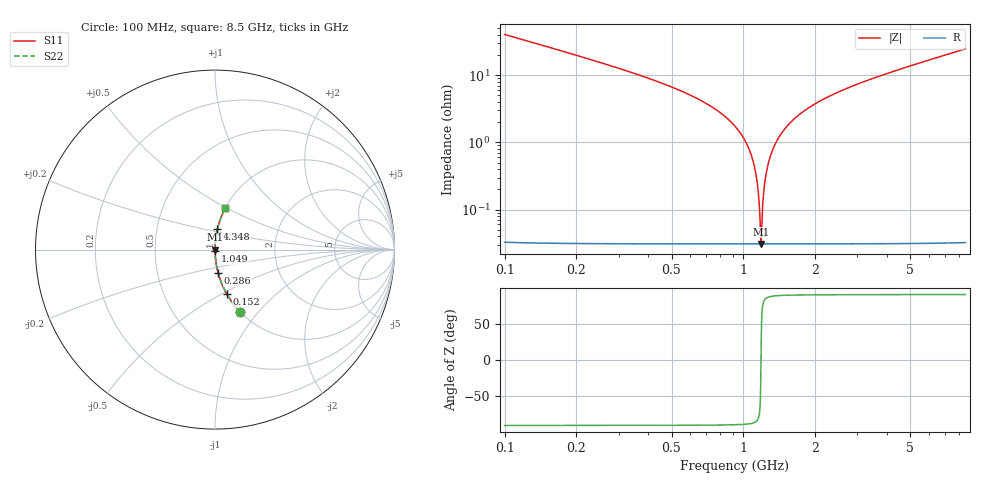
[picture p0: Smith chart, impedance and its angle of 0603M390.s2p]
! Created Wed Apr 18 16:49:37 2012
# hz S ma R 50
! 2 Port Network Data from SP1.SP block
! freq  magS11  angS11  magS21  angS21  magS12  angS12  magS22  angS22
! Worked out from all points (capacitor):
!   8401 points, 100 MHz to 8.5 GHz, reference 50 ohm
!   read as one part in series: C = 39.1 pF near 142 MHz
!   lowest |Z| = 30.9 mohm at 1.185 GHz (marker M1)
!   series resonance near 1.185 GHz, so ESL is about 460 pH
!   S11 on the Smith chart (normalised r, x): 100 MHz: 1.00, -0.81; 152 MHz: 1.00, -0.53; 286 MHz: 1.00, -0.27; 1.049 GHz: 1.00, -0.02; 4.348 GHz: 1.00, +0.23; 8.5 GHz: 1.00, +0.49
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1e8  0.3742 -68.0  0.9271 22.0  0.9271 22.0  0.3742 -68.0
1.52e8  0.2543 -75.2  0.9668 14.7  0.9668 14.7  0.2543 -75.2
2.86e8  0.1326 -82.2  0.9909 7.6  0.9909 7.6  0.1326 -82.2
8.45e8  0.02362 -87.9  0.9994 1.4  0.9994 1.4  0.02362 -87.9
1.049e9  0.008369 -87.4  0.9997 0.5  0.9997 0.5  0.008369 -87.4
1.107e9  0.004663 -85.9  0.9997 0.3  0.9997 0.3  0.004663 -85.9
1.129e9  0.003314 -84.5  0.9997 0.2  0.9997 0.2  0.003314 -84.5
1.157e9  0.001646 -79.1  0.9997 0.1  0.9997 0.1  0.001646 -79.1
1.185e9  0.0003089 4.5  0.9997 -0.0  0.9997 -0.0  0.0003089 4.5
1.21e9  0.001489 78.0  0.9997 -0.1  0.9997 -0.1  0.001489 78.0
1.251e9  0.003759 85.1  0.9997 -0.2  0.9997 -0.2  0.003759 85.1
1.301e9  0.006452 86.9  0.9997 -0.4  0.9997 -0.4  0.006452 86.9
1.383e9  0.01068 87.7  0.9996 -0.6  0.9996 -0.6  0.01068 87.7
1.5e9  0.01636 88.0  0.9996 -0.9  0.9996 -0.9  0.01636 88.0
1.71e9  0.02577 87.8  0.9994 -1.5  0.9994 -1.5  0.02577 87.8
2.001e9  0.03766 87.4  0.999 -2.2  0.999 -2.2  0.03766 87.4
2.9e9  0.06996 85.7  0.9972 -4.0  0.9972 -4.0  0.06996 85.7
4.3e9  0.1149 83.2  0.9931 -6.6  0.9931 -6.6  0.1149 83.2
4.348e9  0.1164 83.2  0.9929 -6.7  0.9929 -6.7  0.1164 83.2
5.7e9  0.1573 80.8  0.9872 -9.1  0.9872 -9.1  0.1573 80.8
7.1e9  0.1987 78.5  0.9798 -11.5  0.9798 -11.5  0.1987 78.5
8.5e9  0.2393 76.1  0.9706 -13.8  0.9706 -13.8  0.2393 76.1
